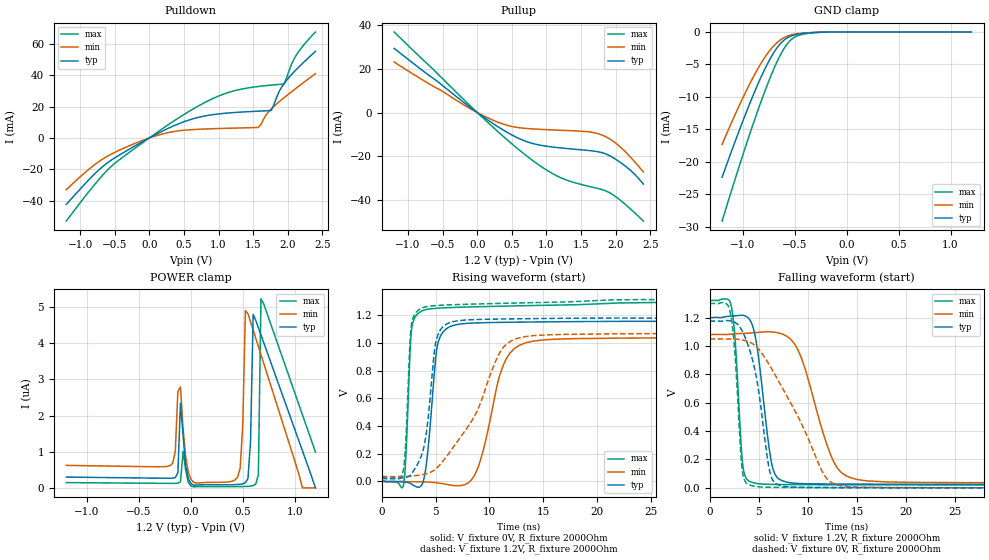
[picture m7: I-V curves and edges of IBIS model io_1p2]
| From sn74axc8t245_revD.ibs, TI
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|   io_1p2 Model
[Model]   io_1p2
Model_type   I/O
Polarity   Non-Inverting
Enable   Active-High
Vinl =  0.360V
Vinh =  0.840V
Vmeas = 0.65
Vref = 0
Cref = 2pF
Rref = 100000
|   typ   min   max
C_comp   1.540pF   1.379pF   1.785pF
| Where Nom  PVT is Nominal Process, 1.2V,  27C
|   Fast PVT is Strong Process,  1.08V, -40C
|   Slow PVT is Weak Process,   1.32V, 130C
[Voltage Range]   1.2   1.08   1.32
|Junction Temperature
[Temperature Range]   27   125   -40
[Pullup Reference]   1.2   1.08   1.32
[Pulldown Reference]   0   0   0
[Power Clamp Reference]   1.2   1.08   1.32
[GND Clamp Reference]   0   0   0
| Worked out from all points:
|   slope of the pulldown table from 0 to 0.18 V, typ, clamps not added: 43.4 ohm
|   slope of the pullup table from 0 to 0.18 V, typ, clamps not added: 44.9 ohm
|   GND clamp passes 1 mA (typ) near -0.58 V on its own axis
|   falling waveform, V_fixture 1.2V, R_fixture 2000Ohm: 20-80 % time 1.22ns typ, 2.7ns min, 653ps max; typ from 1.2 V to 0.025 V
|   rising waveform, V_fixture 0V, R_fixture 2000Ohm: 20-80 % time 779ps typ, 1.84ns min, 414ps max; typ from 0 V to 1.17 V
|   rising waveform, V_fixture 1.2V, R_fixture 2000Ohm: 20-80 % time 984ps typ, 3.88ns min, 438ps max; typ from 0.025 V to 1.2 V
|   falling waveform, V_fixture 0V, R_fixture 2000Ohm: 20-80 % time 1.62ns typ, 4.55ns min, 692ps max; typ from 1.17 V to 0 V
[Pulldown]
|Voltage   I(typ)   I(min)   I(max)
-1.2V     -42.48mA   -33.02mA   -53.03mA
-830mV    -24.74mA   -18.46mA   -31.89mA
-571mV    -14.79mA   -10.84mA   -19.01mA
280mV     6.27mA     3.467mA    8.624mA
650mV     12.46mA    5.369mA    18.91mA
983mV     15.21mA    5.971mA    26.4mA
1.575V    17.08mA    6.668mA    32.84mA
1.76V     17.47mA    18.49mA    33.71mA
1.871V    29.26mA    22.92mA    34.13mA
1.945V    34.64mA    25.61mA    34.37mA
2.13V     43.93mA    32.05mA    53.36mA
2.4V      55.21mA    40.97mA    67.58mA
[GND Clamp]
|Voltage   I(typ)   I(min)   I(max)
-1.2V     -22.38mA   -17.31mA   -29.14mA
-1.075V   -16.88mA   -12.73mA   -22.69mA
-950mV    -11.68mA   -8.497mA   -16.5mA
-850mV    -7.838mA   -5.493mA   -11.83mA
-775mV    -5.268mA   -3.579mA   -8.565mA
-700mV    -3.113mA   -2.076mA   -5.605mA
-625mV    -1.561mA   -1.066mA   -3.12mA
-575mV    -920.5uA   -654.6uA   -1.868mA
-525mV    -552uA     -401.8uA   -1.034mA
-425mV    -234.6uA   -164uA     -348.1uA
-225mV    -22.14uA   -17.06uA   -25.5uA
1.2V      0A         0A         0A
[Pullup]
|Voltage   I(typ)   I(min)   I(max)
-1.2V     29.19mA    22.99mA    36.64mA
106mV     -2.394mA   -1.716mA   -3.142mA
439mV     -9.135mA   -5.863mA   -12.6mA
772mV     -13.83mA   -7.389mA   -21.15mA
994mV     -15.3mA    -7.781mA   -26.02mA
1.216V    -16.14mA   -8.083mA   -29.78mA
1.623V    -17.33mA   -8.841mA   -33.68mA
1.808V    -18.31mA   -10.32mA   -35.1mA
1.919V    -19.78mA   -12.11mA   -36.61mA
2.067V    -22.7mA    -15.69mA   -39.92mA
2.252V    -27.43mA   -21.62mA   -44.98mA
2.4V      -32.57mA   -27.03mA   -49.37mA
[POWER Clamp]
|   Voltage   I(typ)   I(min)   I(max)
-1.2V     298.2nA    621.6nA    145.1nA
-200mV    266.1nA    616nA      123.4nA
-100mV    2.341uA    2.79uA     168.8nA
0V        118.3nA    238.2nA    51.34nA
425mV     88.99nA    217.6nA    34.54nA
475mV     98.89nA    549.3nA    35.51nA
525mV     144.1nA    4.902uA    38.32nA
575mV     1.304uA    4.589uA    48.09nA
600mV     4.796uA    4.364uA    62.93nA
650mV     4.431uA    3.912uA    359.3nA
675mV     4.23uA     3.686uA    5.227uA
1.2V      0A         0A         989.8nA
[Ramp]
R_load = 3000
|   typ   min   max
dV/dt_r   0.617/0.884n   0.530/2.347n   0.709/0.444n
dV/dt_f   0.630/1.551n   0.516/4.264n   0.716/0.748n
[Falling Waveform]
V_fixture = 1.2V
V_fixture_min = 1.08V
V_fixture_max = 1.32V
R_fixture = 2000Ohm
C_fixture = 0F
|   Time   V(typ)   V(min)   V(max)
0s        1.2V       1.08V      1.32V
2.215ns   1.21V      1.083V     1.276V
3.356ns   1.216V     1.088V     171.8mV
4.067ns   1.186V     1.09V      45.69mV
4.807ns   1.001V     1.094V     30.59mV
6.308ns   174.8mV    1.098V     24.69mV
7.487ns   47.71mV    1.081V     23.65mV
12.66ns   27.04mV    181.3mV    21.82mV
14.35ns   26.52mV    71.57mV    21.55mV
50ns      24.68mV    35.54mV    20.57mV
[Rising Waveform]
|Gnd
V_fixture = 0V
V_fixture_min = 0V
V_fixture_max = 0V
R_fixture = 2000Ohm
C_fixture = 0F
|   Time   V(typ)   V(min)   V(max)
0s        133.7nV    980.6nV    44.63nV
2.009ns   -4.057mV   -642.8uV   -30.12mV
2.791ns   -20.07mV   -2.278mV   1.108V
3.93ns    22.29mV    -3.91mV    1.236V
5.182ns   983.9mV    -10.62mV   1.25V
6.831ns   1.13V      -31.19mV   1.256V
8.606ns   1.143V     41.86mV    1.26V
11.28ns   1.148V     836.2mV    1.265V
13.31ns   1.15V      998.6mV    1.268V
50ns      1.17V      1.025V     1.295V
[Rising Waveform]
V_fixture = 1.2V
V_fixture_min = 1.08V
V_fixture_max = 1.32V
R_fixture = 2000Ohm
C_fixture = 0F
|   Time   V(typ)   V(min)   V(max)
0s        24.51mV    35.15mV    20.48mV
1.943ns   26.19mV    35.21mV    57.33mV
2.222ns   29.04mV    34.51mV    270mV
2.748ns   52.31mV    37.91mV    1.126V
3.833ns   221.2mV    49.48mV    1.254V
5.024ns   1.005V     89.9mV     1.269V
6.561ns   1.152V     236.6mV    1.275V
10.91ns   1.171V     920.7mV    1.284V
12.58ns   1.173V     1.032V     1.287V
50ns      1.196V     1.043V     1.317V
[Falling Waveform]
V_fixture = 0V
V_fixture_min = 0V
V_fixture_max = 0V
R_fixture = 2000Ohm
C_fixture = 0F
|   Time   V(typ)   V(min)   V(max)
0s        1.174V     1.049V     1.298V
2.087ns   1.176V     1.049V     1.24V
2.527ns   1.167V     1.049V     988.1mV
3.286ns   1.108V     1.042V     147.3mV
3.989ns   989.8mV    1.029V     22.19mV
6.118ns   116.7mV    861.7mV    4.142mV
6.97ns    21.65mV    757.9mV    3.387mV
11.54ns   2.634mV    105.3mV    1.557mV
13.23ns   2.13mV     16.01mV    1.221mV
50ns      172.5uV    358.9uV    97.61uV
